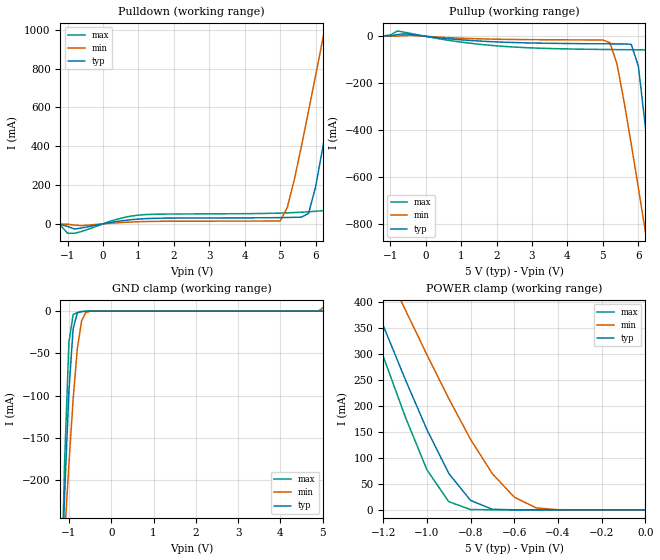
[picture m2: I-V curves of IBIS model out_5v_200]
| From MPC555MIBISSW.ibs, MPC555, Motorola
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| OUTPUT_5v_200(200ns slew rate & operating in Normal mode)
[Model]   out_5v_200
Model_type   Output
Polarity   Non-Inverting
|   typ   min   max
C_comp   5.4970e-13   4.9100e-13   6.2770e-13
| CAP models
| typical : model= typ
| maximum : model= wcs
| minimum : model= bcs
[Voltage range]   5.0v   4.5v   5.5v
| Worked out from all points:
|   slope of the pulldown table from 0 to 0.75 V, typ, clamps not added: 36.8 ohm
|   slope of the pullup table from 0 to 0.75 V, typ, clamps not added: 64.3 ohm
|   GND clamp passes 1 mA (typ) near -0.74 V on its own axis
|   POWER clamp passes 1 mA (typ) near -0.69 V on its own axis
|  typical: model = typ,  temp = 25,  vdd = 5.0
|  maximum: model = bcs,  temp = -40, vdd = 5.5
|  minimum: model = wcs,  temp = 150, vdd = 4.5
[Pulldown]
|  Voltage   I(typ)   I(min)   I(max)
-5V       -240uA     -80uA      -490uA
-1.4V     -1.679mA   -560uA     -3.107mA
-800mV    -26.75mA   -6.541mA   -48.84mA
1V        24.56mA    10.89mA    44.97mA
5V        32.25mA    14.78mA    55.47mA
5.2V      32.85mA    84.21mA    56.67mA
5.8V      53.76mA    581.1mA    62.16mA
6.2V      392.7mA    951.3mA    67.83mA
6.4V      606.4mA    1.139A     86.87mA
6.8V      1.046A     1.517A     494.6mA
7.2V      1.492A     1.899A     1A
10V       4.688A     4.599A     4.7A
[GND_clamp]
-5V       -6.334A    -4.03A     -9.36A
-1.2V     -354.9mA   -354mA     -376.6mA
-1.1V     -215.9mA   -265.7mA   -175.7mA
-1V       -94.26mA   -181.2mA   -36.97mA
-900mV    -20.69mA   -104.3mA   -4.015mA
-800mV    -2.02mA    -44.01mA   -1.604mA
-700mV    -441.8uA   -11.54mA   -531.8uA
-600mV    -101.1uA   -1.48mA    -71.66uA
-500mV    -12.93uA   -156.5uA   -2.926uA
4.8V      63.3pA     19.09uA    56.07pA
4.9V      65.68pA    287.6uA    58.28pA
5V        68.4pA     3.8mA      60.49pA
[Pullup]
-5V       180uA      114uA      247uA
-800mV    7.533mA    1.073mA    22.78mA
5.2V      -32.01mA   -27.27mA   -56.34mA
5.4V      -32.18mA   -120.1mA   -56.64mA
5.8V      -34.51mA   -460.7mA   -57.17mA
6V        -126.9mA   -646.2mA   -57.41mA
6.2V      -387.7mA   -835mA     -58.16mA
6.4V      -683.7mA   -1.026A    -61.86mA
6.6V      -989.5mA   -1.218A    -233.8mA
6.8V      -1.3A      -1.411A    -653.1mA
7V        -1.612A    -1.604A    -1.108A
10V       -6.37A     -4.537A    -8.229A
[POWER_clamp]
-5V       4.559A     4.065A     5.11A
-1.3V     459.2mA    564.9mA    415.1mA
-1.2V     354.1mA    474.5mA    295.2mA
-1.1V     251.6mA    385.3mA    179.8mA
-1V       154.2mA    298mA      77.05mA
-900mV    70.04mA    213.8mA    15.71mA
-800mV    18.08mA    135.3mA    606.6uA
-700mV    1.079mA    69.19mA    104.9uA
-600mV    34.26uA    24.39mA    21.06uA
-500mV    2.117uA    3.8mA      1.676uA
-400mV    134.1nA    287.6uA    45.91nA
0V        68.4pA     5.56nA     71.6pA
| RAMP models
| typical dv/dt : model=typ, temp=25
| maximum dv/dt : model=bcs, temp=-40
| minimum dv/dt : model=wcs, temp=150
|		 typ   min   max
[Ramp]
dV/dt_r   2.1036/1.31415E-09   1.25195/2.75047E-09   3.42681/7.06095E-10
dV/dt_f   2.1036/2.35796E-09   1.25195/4.94916E-09   3.42681/1.05302E-09
